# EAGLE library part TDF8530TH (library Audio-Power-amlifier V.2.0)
The TDF8530 is a quad Bridge-Tied Load (BTL) car audio amplifier comprising an NDMOST-NDMOST output stage based on SOI BCDMOS technology. Low power dissipation enables the TDF8530 high-efficiency, class-D amplifier to be used with a smaller heat sink than those normally used with standard class-AB amplifiers. The TDF8530 can operate in either non-I2C-bus mode or I2C-bus mode. When in I2C-bus mode, DC load detection results and fault conditions can be easily read back from the device. Up to 12 I2C-bus addresses can be selected depending on the value of the external resistors connected to pins ADS and MOD. When pin ADS is short circuited to ground, the TDF8530 operates in non-I2C-bus mode. Switching between Operating mode and Mute mode in non-I2C-bus mode is only possible using pins EN and SEL_MUTE.
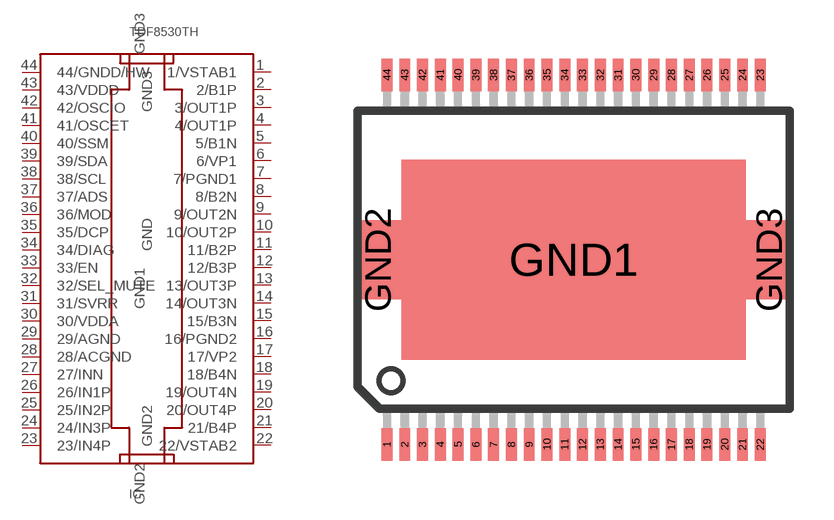
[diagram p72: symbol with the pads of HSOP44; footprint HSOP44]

Designator prefix IC

## TDF8530TH  [HSOP44]
1  1/VSTAB1
2  2/B1P
3  3/OUT1P  out
4  4/OUT1P  out
5  5/B1N
6  6/VP1  pwr
7  7/PGND1  pwr
8  8/B2N
9  9/OUT2N  out
10  10/OUT2P  out
11  11/B2P
12  12/B3P
13  13/OUT3P  out
14  14/OUT3N  out
15  15/B3N
16  16/PGND2  pwr
17  17/VP2  pwr
18  18/B4N
19  19/OUT4N  out
20  20/OUT4P  out
21  21/B4P
22  22/VSTAB2
23  23/IN4P  in
24  24/IN3P  in
25  25/IN2P  in
26  26/IN1P  in
27  27/INN
28  28/ACGND  pwr
29  29/AGND  pwr
30  30/VDDA  pwr
31  31/SVRR
32  32/SEL_MUTE
33  33/EN
34  34/DIAG
35  35/DCP
36  36/MOD
37  37/ADS
38  38/SCL
39  39/SDA
40  40/SSM
41  41/OSCET
42  42/OSCIO
43  43/VDDD  pwr
44  44/GNDD/HW  pwr
GND1  GND  pwr
GND2  GND2
GND3  GND3

## Footprint HSOP44 (pad centres in mm)
44 LEAD HSOP W/PROTRUDING HEADSINK Source: http://www.freescale.com/files/shared/doc/package_info/98ARH98330A.pdf
smd 0.4 x 1.2: 1 -6.825,-6.75; 2 -6.175,-6.75; 3 -5.525,-6.75; 4 -4.875,-6.75; 5 -4.225,-6.75; 6 -3.575,-6.75; 7 -2.925,-6.75; 8 -2.275,-6.75; 9 -1.625,-6.75; 10 -0.975,-6.75; 11 -0.325,-6.75; 12 0.325,-6.75; 13 0.975,-6.75; 14 1.625,-6.75; 15 2.275,-6.75; 16 2.925,-6.75; 17 3.575,-6.75; 18 4.225,-6.75; 19 4.875,-6.75; 20 5.525,-6.75; 21 6.175,-6.75; 22 6.825,-6.75; 23 6.825,6.75; 24 6.175,6.75; 25 5.525,6.75; 26 4.875,6.75; 27 4.225,6.75; 28 3.575,6.75; 29 2.925,6.75; 30 2.275,6.75; 31 1.625,6.75; 32 0.975,6.75; 33 0.325,6.75; 34 -0.325,6.75; 35 -0.975,6.75; 36 -1.625,6.75; 37 -2.275,6.75; 38 -2.925,6.75; 39 -3.575,6.75; 40 -4.225,6.75; 41 -4.875,6.75; 42 -5.525,6.75; 43 -6.175,6.75; 44 -6.825,6.75
smd 12.6 x 7.3: GND1 0,0
smd 1.7 x 2.9: GND2 -7.15,0; GND3 7.15,0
